| IBIS file stm32f7x2_lqfp176.ibs
[IBIS ver] 4.2
[File name] stm32f7x2_lqfp176.ibs
[File Rev] 1.1
[Date]  21-12-2016
[Source] Data Created at STMicroelectronics
[Notes]  File originated from ELDO simulations.
[Disclaimer]  This information is for modeling purpose only and is
   not guaranted.
   The information is subject to change without notice.
[Copyright] Copyright 2017 STMicroelectronics Inc.
|   Component stm32f7x2_lqfp176
[Component] stm32f7x2_lqfp176
[Manufacturer] STMicroelectronics
[Package]
| variable   typ   min   max
R_pkg   0.0   0.0   0.0
L_pkg   0.0H   0.0H   0.0H
C_pkg   0.0F   0.0F   0.0F
[Pin]  signal_name   model_name   R_pin   L_pin   C_pin
1 PE2 io8p_arsudq_ft 235.000E-3 11.500E-9 327.000E-15
2 PE3 io8p_arsudq_ft 229.900E-3 11.200E-9 303.300E-15
3 PE4 io8p_arsudq_ft 225.000E-3 10.800E-9 280.800E-15
4 PE5 io8p_arsudq_ft 220.400E-3 10.500E-9 259.500E-15
5 PE6 io8p_arsudq_ft 216.000E-3 10.300E-9 239.300E-15
6 VBAT power 211.900E-3 10.000E-9 220.200E-15
7 PI8 io8p_arsudq_ft_v33 208.100E-3 9.700E-9 202.300E-15
8 PC13 io8p_arwsudq_ft_v33 204.400E-3 9.500E-9 185.600E-15
9 PC14-OSC32_IN io8p_arwsudq_ft_v33 201.100E-3 9.300E-9 170.000E-15
10 PC15-OSC32_OUT io8p_arwsudq_ft 198.000E-3 9.100E-9 155.600E-15
11 PI9 io8p_arsudq_ft 195.100E-3 8.900E-9 142.300E-15
12 PI10 io8p_arsudq_ft 192.500E-3 8.700E-9 130.200E-15
13 PI11 io8p_arsudq_ft_v33 190.100E-3 8.600E-9 119.200E-15
14 VSS gnd 188.000E-3 8.400E-9 109.400E-15
15 VDD power 186.100E-3 8.300E-9 100.800E-15
16 PF0 io8p_arsudq_i2c_ft 184.500E-3 8.200E-9 93.300E-15
17 PF1 io8p_arsudq_i2c_ft 183.100E-3 8.100E-9 86.900E-15
18 PF2 io8p_arsudq_ft 182.000E-3 8.000E-9 81.700E-15
19 PF3 io8p_arwsudq_ft 181.100E-3 8.000E-9 77.700E-15
20 PF4 io8p_arwsudq_ft 180.500E-3 7.900E-9 74.800E-15
21 PF5 io8p_arwsudq_ft 180.100E-3 7.900E-9 73.100E-15
22 VSS gnd 180.000E-3 7.900E-9 72.500E-15
23 VDD power 180.000E-3 7.900E-9 72.500E-15
24 PF6 io8p_arwsudq_ft 180.100E-3 7.900E-9 73.100E-15
25 PF7 io8p_arwsudq_ft 180.500E-3 7.900E-9 74.800E-15
26 PF8 io8p_arwsudq_ft 181.100E-3 8.000E-9 77.700E-15
27 PF9 io8p_arwsudq_ft 182.000E-3 8.000E-9 81.700E-15
28 PF10 io8p_arwsudq_ft 183.100E-3 8.100E-9 86.900E-15
29 PH0-OSC_IN io8p_arsudq_ft 184.500E-3 8.200E-9 93.300E-15
30 PH1-OSC_OUT io8p_arsudq_ft 186.100E-3 8.300E-9 100.800E-15
31 NRST ioreset_ft_v33 188.000E-3 8.400E-9 109.400E-15
32 PC0 io8p_ar3wsudq_ft 190.100E-3 8.600E-9 119.200E-15
33 PC1 io8p_ar3wsudq_ft_v33 192.500E-3 8.700E-9 130.200E-15
34 PC2 io8p_ar3wsudq_ft 195.100E-3 8.900E-9 142.300E-15
35 PC3 io8p_ar3wsudq_ft 198.000E-3 9.100E-9 155.600E-15
36 VDD power 201.100E-3 9.300E-9 170.000E-15
37 VSSA gnd 204.400E-3 9.500E-9 185.600E-15
38 VREF+ power 208.100E-3 9.700E-9 202.300E-15
39 VDDA power 211.900E-3 10.000E-9 220.200E-15
40 PA0-WKUP io8p_ar3wsudq_ft_v33 216.000E-3 10.300E-9 239.300E-15
41 PA1 io8p_ar3wsudq_ft 220.400E-3 10.500E-9 259.500E-15
42 PA2 io8p_ar3wsudq_ft_v33 225.000E-3 10.800E-9 280.800E-15
43 PH2 io8p_arsudq_ft 229.900E-3 11.200E-9 303.300E-15
44 PH3 io8p_arsudq_ft 235.000E-3 11.500E-9 327.000E-15
45 PH4 io8p_arsudq_i2c_ft 235.000E-3 11.500E-9 327.000E-15
46 PH5 io8p_arsudq_i2c_ft 229.900E-3 11.200E-9 303.300E-15
47 PA3 io8p_ar3wsudq_ft 225.000E-3 10.800E-9 280.800E-15
48 BYPASS_REG gnd 220.400E-3 10.500E-9 259.500E-15
49 VDD power 216.000E-3 10.300E-9 239.300E-15
50 PA4 io8p_ar3wsudq_ft 211.900E-3 10.000E-9 220.200E-15
51 PA5 io8p_ar3wsudq_ft 208.100E-3 9.700E-9 202.300E-15
52 PA6 io8p_ar3wsudq_ft 204.400E-3 9.500E-9 185.600E-15
53 PA7 io8p_ar3wsudq_ft 201.100E-3 9.300E-9 170.000E-15
54 PC4 io8p_ar3wsudq_ft 198.000E-3 9.100E-9 155.600E-15
55 PC5 io8p_ar3wsudq_ft 195.100E-3 8.900E-9 142.300E-15
56 PB0 io8p_ar3wsudq_ft 192.500E-3 8.700E-9 130.200E-15
57 PB1 io8p_ar3wsudq_ft 190.100E-3 8.600E-9 119.200E-15
58 PB2 io8p_ar3wsudq_ft 188.000E-3 8.400E-9 109.400E-15
59 PF11 io8p_arsudq_ft 186.100E-3 8.300E-9 100.800E-15
60 PF12 io8p_arsudq_ft 184.500E-3 8.200E-9 93.300E-15
61 VSS gnd 183.100E-3 8.100E-9 86.900E-15
62 VDD power 182.000E-3 8.000E-9 81.700E-15
63 PF13 io8p_arsudq_ft 181.100E-3 8.000E-9 77.700E-15
64 PF14 io8p_arsudq_ft 180.500E-3 7.900E-9 74.800E-15
65 PF15 io8p_arsudq_ft 180.100E-3 7.900E-9 73.100E-15
66 PG0 io8p_arsudq_ft 180.000E-3 7.900E-9 72.500E-15
67 PG1 io8p_arsudq_ft 180.000E-3 7.900E-9 72.500E-15
68 PE7 io8p_arsudq_ft 180.100E-3 7.900E-9 73.100E-15
69 PE8 io8p_arsudq_ft 180.500E-3 7.900E-9 74.800E-15
70 PE9 io8p_arsudq_ft 181.100E-3 8.000E-9 77.700E-15
71 VSS gnd 182.000E-3 8.000E-9 81.700E-15
72 VDD power 183.100E-3 8.100E-9 86.900E-15
73 PE10 io8p_arsudq_ft 184.500E-3 8.200E-9 93.300E-15
74 PE11 io8p_arsudq_ft 186.100E-3 8.300E-9 100.800E-15
75 PE12 io8p_arsudq_ft 188.000E-3 8.400E-9 109.400E-15
76 PE13 io8p_arsudq_ft 190.100E-3 8.600E-9 119.200E-15
77 PE14 io8p_arsudq_ft 192.500E-3 8.700E-9 130.200E-15
78 PE15 io8p_ar3wsudq_ft 195.100E-3 8.900E-9 142.300E-15
79 PB10 io8p_arsudq_i2c_ft 198.000E-3 9.100E-9 155.600E-15
80 PB11 io8p_arsudq_i2c_ft 201.100E-3 9.300E-9 170.000E-15
81 VCAP_1 power 204.400E-3 9.500E-9 185.600E-15
82 VDD power 208.100E-3 9.700E-9 202.300E-15
83 PH6 io8p_arsudq_ft 211.900E-3 10.000E-9 220.200E-15
84 PH7 io8p_arsudq_i2c_ft 216.000E-3 10.300E-9 239.300E-15
85 PH8 io8p_arsudq_i2c_ft 220.400E-3 10.500E-9 259.500E-15
86 PH9 io8p_arsudq_ft 225.000E-3 10.800E-9 280.800E-15
87 PH10 io8p_arsudq_ft 229.900E-3 11.200E-9 303.300E-15
88 PH11 io8p_arsudq_ft 235.000E-3 11.500E-9 327.000E-15
89 PH12 io8p_arsudq_ft 235.000E-3 11.500E-9 327.000E-15
90 VSS gnd 229.900E-3 11.200E-9 303.300E-15
91 VDD power 225.000E-3 10.800E-9 280.800E-15
92 PB12 io8usb_id_otg_ft 220.400E-3 10.500E-9 259.500E-15
93 PB13 io8usb_vbus_otg_ft 216.000E-3 10.300E-9 239.300E-15
94 PB14 io8usb_lsfs_otg_ft 211.900E-3 10.000E-9 220.200E-15
95 PB15 io8usb_lsfs_otg_ft 208.100E-3 9.700E-9 202.300E-15
96 PD8 io8p_arsudq_ft 204.400E-3 9.500E-9 185.600E-15
97 PD9 io8p_arsudq_ft 201.100E-3 9.300E-9 170.000E-15
98 PD10 io8p_arsudq_ft 198.000E-3 9.100E-9 155.600E-15
99 PD11 io8p_arsudq_ft 195.100E-3 8.900E-9 142.300E-15
100 PD12 io8p_arsudq_ft 192.500E-3 8.700E-9 130.200E-15
101 PD13 io8p_arsudq_ft 190.100E-3 8.600E-9 119.200E-15
102 VSS gnd 188.000E-3 8.400E-9 109.400E-15
103 VDD power 186.100E-3 8.300E-9 100.800E-15
104 PD14 io8p_arsudq_ft 184.500E-3 8.200E-9 93.300E-15
105 PD15 io8p_arsudq_ft 183.100E-3 8.100E-9 86.900E-15
106 PG2 io8p_arsudq_ft 182.000E-3 8.000E-9 81.700E-15
107 PG3 io8p_arsudq_ft 181.100E-3 8.000E-9 77.700E-15
108 PG4 io8p_arsudq_ft 180.500E-3 7.900E-9 74.800E-15
109 PG5 io8p_arsudq_ft 180.100E-3 7.900E-9 73.100E-15
110 PG6 io8p_arsudq_ft 180.000E-3 7.900E-9 72.500E-15
111 PG7 io8p_arsudq_ft 180.000E-3 7.900E-9 72.500E-15
112 PG8 io8p_arsudq_ft 180.100E-3 7.900E-9 73.100E-15
113 VSS gnd 180.500E-3 7.900E-9 74.800E-15
114 VDDUSB power 181.100E-3 8.000E-9 77.700E-15
115 PC6 io8p_arsudq_ft 182.000E-3 8.000E-9 81.700E-15
116 PC7 io8p_arsudq_ft 183.100E-3 8.100E-9 86.900E-15
117 PC8 io8p_arsudq_ft 184.500E-3 8.200E-9 93.300E-15
118 PC9 io8p_arsudq_i2c_ft 186.100E-3 8.300E-9 100.800E-15
119 PA8 io8p_arsudq_i2c_ft 188.000E-3 8.400E-9 109.400E-15
120 PA9 io8usb_vbus_otg_ft 190.100E-3 8.600E-9 119.200E-15
121 PA10 io8usb_id_otg_ft 192.500E-3 8.700E-9 130.200E-15
122 PA11 io8usb_lsfs_otg_ft 195.100E-3 8.900E-9 142.300E-15
123 PA12 io8usb_lsfs_otg_ft 198.000E-3 9.100E-9 155.600E-15
124 PA13 io8p_arsudq_ft 201.100E-3 9.300E-9 170.000E-15
125 VCAP_2 power 204.400E-3 9.500E-9 185.600E-15
126 VSS gnd 208.100E-3 9.700E-9 202.300E-15
127 VDD power 211.900E-3 10.000E-9 220.200E-15
128 PH13 io8p_arsudq_ft 216.000E-3 10.300E-9 239.300E-15
129 PH14 io8p_arsudq_ft 220.400E-3 10.500E-9 259.500E-15
130 PH15 io8p_arsudq_ft 225.000E-3 10.800E-9 280.800E-15
131 PI0 io8p_arsudq_ft 229.900E-3 11.200E-9 303.300E-15
132 PI1 io8p_arsudq_ft 235.000E-3 11.500E-9 327.000E-15
133 PI2 io8p_arsudq_ft 235.000E-3 11.500E-9 327.000E-15
134 PI3 io8p_arsudq_ft 229.900E-3 11.200E-9 303.300E-15
135 VSS gnd 225.000E-3 10.800E-9 280.800E-15
136 VDD power 220.400E-3 10.500E-9 259.500E-15
137 PA14 io8p_arsudq_ft 216.000E-3 10.300E-9 239.300E-15
138 PA15 io8p_arsudq_ft 211.900E-3 10.000E-9 220.200E-15
139 PC10 io8p_arsudq_ft 208.100E-3 9.700E-9 202.300E-15
140 PC11 io8p_arsudq_ft 204.400E-3 9.500E-9 185.600E-15
141 PC12 io8p_arsudq_ft 201.100E-3 9.300E-9 170.000E-15
142 PD0 io8p_arsudq_ft 198.000E-3 9.100E-9 155.600E-15
143 PD1 io8p_arsudq_ft 195.100E-3 8.900E-9 142.300E-15
144 PD2 io8p_arsudq_ft 192.500E-3 8.700E-9 130.200E-15
145 PD3 io8p_arsudq_ft 190.100E-3 8.600E-9 119.200E-15
146 PD4 io8p_arsudq_ft 188.000E-3 8.400E-9 109.400E-15
147 PD5 io8p_arsudq_ft 186.100E-3 8.300E-9 100.800E-15
148 VSS gnd 184.500E-3 8.200E-9 93.300E-15
149 VDDSDMMC power 183.100E-3 8.100E-9 86.900E-15
150 PD6 io8p_arsudq_ft 182.000E-3 8.000E-9 81.700E-15
151 PD7 io8p_arsudq_ft 181.100E-3 8.000E-9 77.700E-15
152 PG9 io8p_arsudq_ft 180.500E-3 7.900E-9 74.800E-15
153 PG10 io8p_arsudq_ft 180.100E-3 7.900E-9 73.100E-15
154 PG11 io8p_arsudq_ft 180.000E-3 7.900E-9 72.500E-15
155 PG12 io8p_arsudq_ft 180.000E-3 7.900E-9 72.500E-15
156 PG13 io8p_arsudq_ft 180.100E-3 7.900E-9 73.100E-15
157 PG14 io8p_arsudq_ft 180.500E-3 7.900E-9 74.800E-15
158 VSS gnd 181.100E-3 8.000E-9 77.700E-15
159 VDD power 182.000E-3 8.000E-9 81.700E-15
160 PG15 io8p_arsudq_ft 183.100E-3 8.100E-9 86.900E-15
161 PB3 io8p_arsudq_ft 184.500E-3 8.200E-9 93.300E-15
162 PB4 io8p_arsudq_ft 186.100E-3 8.300E-9 100.800E-15
163 PB5 io8p_ar3wsudq_ft 188.000E-3 8.400E-9 109.400E-15
164 PB6 io8p_arsudq_i2c_ft 190.100E-3 8.600E-9 119.200E-15
165 PB7 io8p_arsudq_i2c_ft 192.500E-3 8.700E-9 130.200E-15
166 BOOT0 vpp_test_hv 195.100E-3 8.900E-9 142.300E-15
167 PB8 io8p_arsudq_i2c_ft 198.000E-3 9.100E-9 155.600E-15
168 PB9 io8p_arsudq_i2c_ft 201.100E-3 9.300E-9 170.000E-15
169 PE0 io8p_arsudq_ft 204.400E-3 9.500E-9 185.600E-15
170 PE1 io8p_arsudq_ft 208.100E-3 9.700E-9 202.300E-15
171 PDR_ON gnd 211.900E-3 10.000E-9 220.200E-15
172 VDD power 216.000E-3 10.300E-9 239.300E-15
173 PI4 io8p_arsudq_ft 220.400E-3 10.500E-9 259.500E-15
174 PI5 io8p_arsudq_ft 225.000E-3 10.800E-9 280.800E-15
175 PI6 io8p_arsudq_ft 229.900E-3 11.200E-9 303.300E-15
176 PI7 io8p_arsudq_ft 235.000E-3 11.500E-9 327.000E-15
[Diff Pin]   inv_pin   vdiff   tdelay_typ  tdelay_min  tdelay_max
94   95   NA   NA   NA   NA
122   123   NA   NA   NA   NA
[Model Selector] io8p_arsudq_ft_v33
io8p00_arsudq_ft_v33_pd_lv  "SPEED00 1P8V, PD=40kOhm"
io8p00_arsudq_ft_v33_pu_lv  "SPEED00 1P8V, PU=40kOhm"
io8p00_arsudq_ft_v33_lv  "SPEED00 1P8V"
io8p01_arsudq_ft_v33_pd_lv  "SPEED01 1P8V, PD=40kOhm"
io8p01_arsudq_ft_v33_pu_lv  "SPEED01 1P8V, PU=40kOhm"
io8p01_arsudq_ft_v33_lv  "SPEED01 1P8V"
io8p10_arsudq_ft_v33_pd_lv  "SPEED10 1P8V, PD=40kOhm"
io8p10_arsudq_ft_v33_pu_lv  "SPEED10 1P8V, PU=40kOhm"
io8p10_arsudq_ft_v33_lv  "SPEED10 1P8V"
io8p11_arsudq_ft_v33_pd_lv  "SPEED11 1P8V, PD=40kOhm"
io8p11_arsudq_ft_v33_pu_lv  "SPEED11 1P8V, PU=40kOhm"
io8p11_arsudq_ft_v33_lv  "SPEED11 1P8V"
io8p00_arsudq_ft_v33_pd  "SPEED00, PD=40kOhm"
io8p00_arsudq_ft_v33_pu  "SPEED00, PU=40kOhm"
io8p00_arsudq_ft_v33  "SPEED00"
io8p01_arsudq_ft_v33_pd  "SPEED01, PD=40kOhm"
io8p01_arsudq_ft_v33_pu  "SPEED01, PU=40kOhm"
io8p01_arsudq_ft_v33  "SPEED01"
io8p10_arsudq_ft_v33_pd  "SPEED10, PD=40kOhm"
io8p10_arsudq_ft_v33_pu  "SPEED10, PU=40kOhm"
io8p10_arsudq_ft_v33  "SPEED10"
io8p11_arsudq_ft_v33_pd  "SPEED11, PD=40kOhm"
io8p11_arsudq_ft_v33_pu  "SPEED11, PU=40kOhm"
io8p11_arsudq_ft_v33  "SPEED11"
[Model Selector] io8p_ar3wsudq_ft
io8p00_ar3wsudq_ft_pd_lv  "SPEED00 1P8V, PD=40kOhm"
io8p00_ar3wsudq_ft_pu_lv  "SPEED00 1P8V, PU=40kOhm"
io8p00_ar3wsudq_ft_lv  "SPEED00 1P8V"
io8p01_ar3wsudq_ft_pd_lv  "SPEED01 1P8V, PD=40kOhm"
io8p01_ar3wsudq_ft_pu_lv  "SPEED01 1P8V, PU=40kOhm"
io8p01_ar3wsudq_ft_lv  "SPEED01 1P8V"
io8p10_ar3wsudq_ft_pd_lv  "SPEED10 1P8V, PD=40kOhm"
io8p10_ar3wsudq_ft_pu_lv  "SPEED10 1P8V, PU=40kOhm"
io8p10_ar3wsudq_ft_lv  "SPEED10 1P8V"
io8p11_ar3wsudq_ft_pd_lv  "SPEED11 1P8V, PD=40kOhm"
io8p11_ar3wsudq_ft_pu_lv  "SPEED11 1P8V, PU=40kOhm"
io8p11_ar3wsudq_ft_lv  "SPEED11 1P8V"
io8p00_ar3wsudq_ft_pd  "SPEED00, PD=40kOhm"
io8p00_ar3wsudq_ft_pu  "SPEED00, PU=40kOhm"
io8p00_ar3wsudq_ft  "SPEED00"
io8p01_ar3wsudq_ft_pd  "SPEED01, PD=40kOhm"
io8p01_ar3wsudq_ft_pu  "SPEED01, PU=40kOhm"
io8p01_ar3wsudq_ft  "SPEED01"
io8p10_ar3wsudq_ft_pd  "SPEED10, PD=40kOhm"
io8p10_ar3wsudq_ft_pu  "SPEED10, PU=40kOhm"
io8p10_ar3wsudq_ft  "SPEED10"
io8p11_ar3wsudq_ft_pd  "SPEED11, PD=40kOhm"
io8p11_ar3wsudq_ft_pu  "SPEED11, PU=40kOhm"
io8p11_ar3wsudq_ft  "SPEED11"
[Model Selector] io8p_ar3wsudq_ft_v33
io8p00_ar3wsudq_ft_v33_pd_lv  "SPEED00 1P8V, PD=40kOhm"
io8p00_ar3wsudq_ft_v33_pu_lv  "SPEED00 1P8V, PU=40kOhm"
io8p00_ar3wsudq_ft_v33_lv  "SPEED00 1P8V"
io8p01_ar3wsudq_ft_v33_pd_lv  "SPEED01 1P8V, PD=40kOhm"
io8p01_ar3wsudq_ft_v33_pu_lv  "SPEED01 1P8V, PU=40kOhm"
io8p01_ar3wsudq_ft_v33_lv  "SPEED01 1P8V"
io8p10_ar3wsudq_ft_v33_pd_lv  "SPEED10 1P8V, PD=40kOhm"
io8p10_ar3wsudq_ft_v33_pu_lv  "SPEED10 1P8V, PU=40kOhm"
io8p10_ar3wsudq_ft_v33_lv  "SPEED10 1P8V"
io8p11_ar3wsudq_ft_v33_pd_lv  "SPEED11 1P8V, PD=40kOhm"
io8p11_ar3wsudq_ft_v33_pu_lv  "SPEED11 1P8V, PU=40kOhm"
io8p11_ar3wsudq_ft_v33_lv  "SPEED11 1P8V"
io8p00_ar3wsudq_ft_v33_pd  "SPEED00, PD=40kOhm"
io8p00_ar3wsudq_ft_v33_pu  "SPEED00, PU=40kOhm"
io8p00_ar3wsudq_ft_v33  "SPEED00"
io8p01_ar3wsudq_ft_v33_pd  "SPEED01, PD=40kOhm"
io8p01_ar3wsudq_ft_v33_pu  "SPEED01, PU=40kOhm"
io8p01_ar3wsudq_ft_v33  "SPEED01"
io8p10_ar3wsudq_ft_v33_pd  "SPEED10, PD=40kOhm"
io8p10_ar3wsudq_ft_v33_pu  "SPEED10, PU=40kOhm"
io8p10_ar3wsudq_ft_v33  "SPEED10"
io8p11_ar3wsudq_ft_v33_pd  "SPEED11, PD=40kOhm"
io8p11_ar3wsudq_ft_v33_pu  "SPEED11, PU=40kOhm"
io8p11_ar3wsudq_ft_v33  "SPEED11"
[Model Selector] io8p_arsudq_ft
io8p00_arsudq_ft_pd_lv  "SPEED00 1P8V, PD=40kOhm"
io8p00_arsudq_ft_pu_lv  "SPEED00 1P8V, PU=40kOhm"
io8p00_arsudq_ft_lv  "SPEED00 1P8V"
io8p01_arsudq_ft_pd_lv  "SPEED01 1P8V, PD=40kOhm"
io8p01_arsudq_ft_pu_lv  "SPEED01 1P8V, PU=40kOhm"
io8p01_arsudq_ft_lv  "SPEED01 1P8V"
io8p10_arsudq_ft_pd_lv  "SPEED10 1P8V, PD=40kOhm"
io8p10_arsudq_ft_pu_lv  "SPEED10 1P8V, PU=40kOhm"
io8p10_arsudq_ft_lv  "SPEED10 1P8V"
io8p11_arsudq_ft_pd_lv  "SPEED11 1P8V, PD=40kOhm"
io8p11_arsudq_ft_pu_lv  "SPEED11 1P8V, PU=40kOhm"
io8p11_arsudq_ft_lv  "SPEED11 1P8V"
io8p00_arsudq_ft_pd  "SPEED00, PD=40kOhm"
io8p00_arsudq_ft_pu  "SPEED00, PU=40kOhm"
io8p00_arsudq_ft  "SPEED00"
io8p01_arsudq_ft_pd  "SPEED01, PD=40kOhm"
io8p01_arsudq_ft_pu  "SPEED01, PU=40kOhm"
io8p01_arsudq_ft  "SPEED01"
io8p10_arsudq_ft_pd  "SPEED10, PD=40kOhm"
io8p10_arsudq_ft_pu  "SPEED10, PU=40kOhm"
io8p10_arsudq_ft  "SPEED10"
io8p11_arsudq_ft_pd  "SPEED11, PD=40kOhm"
io8p11_arsudq_ft_pu  "SPEED11, PU=40kOhm"
io8p11_arsudq_ft  "SPEED11"
[Model Selector] io8p_arsudq_i2c_ft
io8prog_1v8_i2c_pd  "5V Tol GPIO 1.8V range i2c functionality with pull down"
io8prog_1v8_i2c_pu  "5V Tol GPIO 1.8V range i2c functionality with pull up"
io8prog_1v8_i2c  "5V Tol GPIO 1.8V range i2c functionality"
io8prog_3v3_i2c_pd  "5V Tol GPIO 3.3V range i2c functionality with pull down"
io8prog_3v3_i2c_pu  "5V Tol GPIO 3.3V range i2c functionality with pull up"
io8prog_3v3_i2c  "5V Tol GPIO 3.3V range i2c functionality"
io8prog_1v8_pd_00  "5V Tol GPIO 1.8V range with pd speed 00"
io8prog_1v8_pu_00  "5V Tol GPIO 1.8V range with pu speed 00"
io8prog_1v8_00  "5V Tol GPIO 1.8V range speed 00"
io8prog_3v3_pd_00  "5V Tol GPIO 3.3V range with pd speed 00"
io8prog_3v3_pu_00  "5V Tol GPIO 3.3V range with pu speed 00"
io8prog_3v3_00  "5V Tol GPIO 3.3V range speed 00"
io8prog_1v8_pd_01  "5V Tol GPIO 1.8V range with pd speed 01"
io8prog_1v8_pu_01  "5V Tol GPIO 1.8V range with pu speed 01"
io8prog_1v8_01  "5V Tol GPIO 1.8V range speed 01"
io8prog_3v3_pd_01  "5V Tol GPIO 3.3V range with pd speed 01"
io8prog_3v3_pu_01  "5V Tol GPIO 3.3V range with pu speed 01"
io8prog_3v3_01  "5V Tol GPIO 3.3V range speed 01"
io8prog_1v8_pd_10  "5V Tol GPIO 1.8V range with pd speed 10"
io8prog_1v8_pu_10  "5V Tol GPIO 1.8V range with pu speed 10"
io8prog_1v8_10  "5V Tol GPIO 1.8V range speed 10"
io8prog_3v3_pd_10  "5V Tol GPIO 3.3V range with pd speed 10"
io8prog_3v3_pu_10  "5V Tol GPIO 3.3V range with pu speed 10"
io8prog_3v3_10  "5V Tol GPIO 3.3V range speed 10"
io8prog_1v8_pd_11  "5V Tol GPIO 1.8V range with pd speed 11"
io8prog_1v8_pu_11  "5V Tol GPIO 1.8V range with pu speed 11"
io8prog_1v8_11  "5V Tol GPIO 1.8V range speed 11"
io8prog_3v3_pd_11  "5V Tol GPIO 3.3V range with pd speed 11"
io8prog_3v3_pu_11  "5V Tol GPIO 3.3V range with pu speed 11"
io8prog_3v3_11  "5V Tol GPIO 3.3V range speed 11"
[Model Selector] io8p_arwsudq_ft
io8p00_arwsudq_ft_pd_lv  "SPEED00 1P8V, PD=40kOhm"
io8p00_arwsudq_ft_pu_lv  "SPEED00 1P8V, PU=40kOhm"
io8p00_arwsudq_ft_lv  "SPEED00 1P8V"
io8p01_arwsudq_ft_pd_lv  "SPEED01 1P8V, PD=40kOhm"
io8p01_arwsudq_ft_pu_lv  "SPEED01 1P8V, PU=40kOhm"
io8p01_arwsudq_ft_lv  "SPEED01 1P8V"
io8p10_arwsudq_ft_pd_lv  "SPEED10 1P8V, PD=40kOhm"
io8p10_arwsudq_ft_pu_lv  "SPEED10 1P8V, PU=40kOhm"
io8p10_arwsudq_ft_lv  "SPEED10 1P8V"
io8p11_arwsudq_ft_pd_lv  "SPEED11 1P8V, PD=40kOhm"
io8p11_arwsudq_ft_pu_lv  "SPEED11 1P8V, PU=40kOhm"
io8p11_arwsudq_ft_lv  "SPEED11 1P8V"
io8p00_arwsudq_ft_pd  "SPEED00, PD=40kOhm"
io8p00_arwsudq_ft_pu  "SPEED00, PU=40kOhm"
io8p00_arwsudq_ft  "SPEED00"
io8p01_arwsudq_ft_pd  "SPEED01, PD=40kOhm"
io8p01_arwsudq_ft_pu  "SPEED01, PU=40kOhm"
io8p01_arwsudq_ft  "SPEED01"
io8p10_arwsudq_ft_pd  "SPEED10, PD=40kOhm"
io8p10_arwsudq_ft_pu  "SPEED10, PU=40kOhm"
io8p10_arwsudq_ft  "SPEED10"
io8p11_arwsudq_ft_pd  "SPEED11, PD=40kOhm"
io8p11_arwsudq_ft_pu  "SPEED11, PU=40kOhm"
io8p11_arwsudq_ft  "SPEED11"
[Model Selector] io8p_arwsudq_ft_v33
io8p00_arwsudq_ft_v33_pd_lv  "SPEED00 1P8V, PD=40kOhm"
io8p00_arwsudq_ft_v33_pu_lv  "SPEED00 1P8V, PU=40kOhm"
io8p00_arwsudq_ft_v33_lv  "SPEED00 1P8V"
io8p01_arwsudq_ft_v33_pd_lv  "SPEED01 1P8V, PD=40kOhm"
io8p01_arwsudq_ft_v33_pu_lv  "SPEED01 1P8V, PU=40kOhm"
io8p01_arwsudq_ft_v33_lv  "SPEED01 1P8V"
io8p10_arwsudq_ft_v33_pd_lv  "SPEED10 1P8V, PD=40kOhm"
io8p10_arwsudq_ft_v33_pu_lv  "SPEED10 1P8V, PU=40kOhm"
io8p10_arwsudq_ft_v33_lv  "SPEED10 1P8V"
io8p11_arwsudq_ft_v33_pd_lv  "SPEED11 1P8V, PD=40kOhm"
io8p11_arwsudq_ft_v33_pu_lv  "SPEED11 1P8V, PU=40kOhm"
io8p11_arwsudq_ft_v33_lv  "SPEED11 1P8V"
io8p00_arwsudq_ft_v33_pd  "SPEED00, PD=40kOhm"
io8p00_arwsudq_ft_v33_pu  "SPEED00, PU=40kOhm"
io8p00_arwsudq_ft_v33  "SPEED00"
io8p01_arwsudq_ft_v33_pd  "SPEED01, PD=40kOhm"
io8p01_arwsudq_ft_v33_pu  "SPEED01, PU=40kOhm"
io8p01_arwsudq_ft_v33  "SPEED01"
io8p10_arwsudq_ft_v33_pd  "SPEED10, PD=40kOhm"
io8p10_arwsudq_ft_v33_pu  "SPEED10, PU=40kOhm"
io8p10_arwsudq_ft_v33  "SPEED10"
io8p11_arwsudq_ft_v33_pd  "SPEED11, PD=40kOhm"
io8p11_arwsudq_ft_v33_pu  "SPEED11, PU=40kOhm"
io8p11_arwsudq_ft_v33  "SPEED11"
[Model Selector] io8usb_id_otg_ft
io8p00_id_otg_ft_pd_lv  "SPEED00 1P8V, PD=14kOhm"
io8p00_id_otg_ft_pu_lv  "SPEED00 1P8V, PU=14kOhm"
io8p00_id_otg_ft_lv  "SPEED00 1P8V"
io8p01_id_otg_ft_pd_lv  "SPEED01 1P8V, PD=14kOhm"
io8p01_id_otg_ft_pu_lv  "SPEED01 1P8V, PU=14kOhm"
io8p01_id_otg_ft_lv  "SPEED01 1P8V"
io8p10_id_otg_ft_pd_lv  "SPEED10 1P8V, PD=14kOhm"
io8p10_id_otg_ft_pu_lv  "SPEED10 1P8V, PU=14kOhm"
io8p10_id_otg_ft_lv  "SPEED10 1P8V"
io8p11_id_otg_ft_pd_lv  "SPEED11 1P8V, PD=14kOhm"
io8p11_id_otg_ft_pu_lv  "SPEED11 1P8V, PU=14kOhm"
io8p11_id_otg_ft_lv  "SPEED11 1P8V"
io8p00_id_otg_ft_pd  "SPEED00, PD=14kOhm"
io8p00_id_otg_ft_pu  "SPEED00, PU=14kOhm"
io8p00_id_otg_ft  "SPEED00"
io8p01_id_otg_ft_pd  "SPEED01, PD=14kOhm"
io8p01_id_otg_ft_pu  "SPEED01, PU=14kOhm"
io8p01_id_otg_ft  "SPEED01"
io8p10_id_otg_ft_pd  "SPEED10, PD=14kOhm"
io8p10_id_otg_ft_pu  "SPEED10, PU=14kOhm"
io8p10_id_otg_ft  "SPEED10"
io8p11_id_otg_ft_pd  "SPEED11, PD=14kOhm"
io8p11_id_otg_ft_pu  "SPEED11, PU=14kOhm"
io8p11_id_otg_ft  "SPEED11"
[Model Selector] io8usb_lsfs_otg_ft
io8usb_ls_otg_ft_dpdn_pd  "LS USB DP/DN IO + PD=20kOhm"
io8usb_ls_otg_ft_dpdn_pupu2  "LS USB DP/DN IO + PU/PU2=2.2kOhm"
io8usb_ls_otg_ft_dpdn_pu2  "LS USB DP/DN IO + PU2=1.2kOhm"
io8usb_ls_otg_ft_dpdn_pu  "LS USB DP/DN IO + PU=1.2kOhm"
io8usb_ls_otg_ft_dpdn  "LS USB DP/DN IO"
io8usb_fs_otg_ft_dpdn_pd  "HS USB DP/DN IO + PD=20kOhm"
io8usb_fs_otg_ft_dpdn_pupu2  "HS USB DP/DN IO + PU/PU2=2.2kOhm"
io8usb_fs_otg_ft_dpdn_pu2  "HS USB DP/DN IO + PU2=1.2kOhm"
io8usb_fs_otg_ft_dpdn_pu  "HS USB DP/DN IO + PU=1.2kOhm"
io8usb_fs_otg_ft_dpdn  "HS USB DP/DN IO"
io8p00_lsfs_otg_ft_pd_lv  "SPEED00 1P8V, PD=40kOhm"
io8p00_lsfs_otg_ft_pu_lv  "SPEED00 1P8V, PU=40kOhm"
io8p00_lsfs_otg_ft_lv  "SPEED00 1P8V"
io8p01_lsfs_otg_ft_pd_lv  "SPEED01 1P8V, PD=40kOhm"
io8p01_lsfs_otg_ft_pu_lv  "SPEED01 1P8V, PU=40kOhm"
io8p01_lsfs_otg_ft_lv  "SPEED01 1P8V"
io8p10_lsfs_otg_ft_pd_lv  "SPEED10 1P8V, PD=40kOhm"
io8p10_lsfs_otg_ft_pu_lv  "SPEED10 1P8V, PU=40kOhm"
io8p10_lsfs_otg_ft_lv  "SPEED10 1P8V"
io8p11_lsfs_otg_ft_pd_lv  "SPEED11 1P8V, PD=40kOhm"
io8p11_lsfs_otg_ft_pu_lv  "SPEED11 1P8V, PU=40kOhm"
io8p11_lsfs_otg_ft_lv  "SPEED11 1P8V"
io8p00_lsfs_otg_ft_pd  "SPEED00, PD=40kOhm"
io8p00_lsfs_otg_ft_pu  "SPEED00, PU=40kOhm"
io8p00_lsfs_otg_ft  "SPEED00"
io8p01_lsfs_otg_ft_pd  "SPEED01, PD=40kOhm"
io8p01_lsfs_otg_ft_pu  "SPEED01, PU=40kOhm"
io8p01_lsfs_otg_ft  "SPEED01"
io8p10_lsfs_otg_ft_pd  "SPEED10, PD=40kOhm"
io8p10_lsfs_otg_ft_pu  "SPEED10, PU=40kOhm"
io8p10_lsfs_otg_ft  "SPEED10"
io8p11_lsfs_otg_ft_pd  "SPEED11, PD=40kOhm"
io8p11_lsfs_otg_ft_pu  "SPEED11, PU=40kOhm"
io8p11_lsfs_otg_ft  "SPEED11"
[Model Selector] io8usb_vbus_otg_ft
io8psenb_vbus_otg_ft  "VBUS PULSE, SENSE VB"
io8psenab_vbus_otg_ft  "VBUS PULSE, SENSE VA and VB"
io8psena_vbus_otg_ft  "VBUS PULSE, SENSE VA"
io8psen_vbus_otg_ft  "VBUS PULSE"
io8p00_vbus_otg_ft_pd_lv  "SPEED00 1P8V, PD=40kOhm"
io8p00_vbus_otg_ft_pu_lv  "SPEED00 1P8V, PU=40kOhm"
io8p00_vbus_otg_ft_lv  "SPEED00 1P8V"
io8p01_vbus_otg_ft_pd_lv  "SPEED01 1P8V, PD=40kOhm"
io8p01_vbus_otg_ft_pu_lv  "SPEED01 1P8V, PU=40kOhm"
io8p01_vbus_otg_ft_lv  "SPEED01 1P8V"
io8p10_vbus_otg_ft_pd_lv  "SPEED10 1P8V, PD=40kOhm"
io8p10_vbus_otg_ft_pu_lv  "SPEED10 1P8V, PU=40kOhm"
io8p10_vbus_otg_ft_lv  "SPEED10 1P8V"
io8p11_vbus_otg_ft_pd_lv  "SPEED11 1P8V, PD=40kOhm"
io8p11_vbus_otg_ft_pu_lv  "SPEED11 1P8V, PU=40kOhm"
io8p11_vbus_otg_ft_lv  "SPEED11 1P8V"
io8p00_vbus_otg_ft_pd  "SPEED00, PD=40kOhm"
io8p00_vbus_otg_ft_pu  "SPEED00, PU=40kOhm"
io8p00_vbus_otg_ft  "SPEED00"
io8p01_vbus_otg_ft_pd  "SPEED01, PD=40kOhm"
io8p01_vbus_otg_ft_pu  "SPEED01, PU=40kOhm"
io8p01_vbus_otg_ft  "SPEED01"
io8p10_vbus_otg_ft_pd  "SPEED10, PD=40kOhm"
io8p10_vbus_otg_ft_pu  "SPEED10, PU=40kOhm"
io8p10_vbus_otg_ft  "SPEED10"
io8p11_vbus_otg_ft_pd  "SPEED11, PD=40kOhm"
io8p11_vbus_otg_ft_pu  "SPEED11, PU=40kOhm"
io8p11_vbus_otg_ft  "SPEED11"
[Model Selector] ioreset_ft_v33
ioreset_ft_v33_pu_lv  "IORESET 1P8V + PU=40kOhm"
ioreset_ft_v33_nopu_lv  "IORESET 1P8V"
ioreset_ft_v33_pu  "IORESET + PU=40kOhm"
ioreset_ft_v33_nopu  "IORESET"
[Model Selector] vpp_test_hv
vpp_test_hv_2p4  "Input Buffer 1P8V"
vpp_test_hv_3p3  "Input Buffer"
| Models and submodels in the file (266): io8p00_arsudq_ft_v33_pd_lv (I/O), io8p00_arsudq_ft_v33_pu_lv (I/O), io8p00_arsudq_ft_v33_lv (I/O), io8p01_arsudq_ft_v33_pd_lv (I/O), io8p01_arsudq_ft_v33_pu_lv (I/O), io8p01_arsudq_ft_v33_lv (I/O), io8p10_arsudq_ft_v33_pd_lv (I/O), io8p10_arsudq_ft_v33_pu_lv (I/O), io8p10_arsudq_ft_v33_lv (I/O), io8p11_arsudq_ft_v33_pd_lv (I/O), io8p11_arsudq_ft_v33_pu_lv (I/O), io8p11_arsudq_ft_v33_lv (I/O), io8p00_arsudq_ft_v33_pd (I/O), io8p00_arsudq_ft_v33_pu (I/O), io8p00_arsudq_ft_v33 (I/O), io8p01_arsudq_ft_v33_pd (I/O), io8p01_arsudq_ft_v33_pu (I/O), io8p01_arsudq_ft_v33 (I/O), io8p10_arsudq_ft_v33_pd (I/O), io8p10_arsudq_ft_v33_pu (I/O), io8p10_arsudq_ft_v33 (I/O), io8p11_arsudq_ft_v33_pd (I/O), io8p11_arsudq_ft_v33_pu (I/O), io8p11_arsudq_ft_v33 (I/O), io8p00_ar3wsudq_ft_pd_lv (I/O), io8p00_ar3wsudq_ft_pu_lv (I/O), io8p00_ar3wsudq_ft_lv (I/O), io8p01_ar3wsudq_ft_pd_lv (I/O), io8p01_ar3wsudq_ft_pu_lv (I/O), io8p01_ar3wsudq_ft_lv (I/O), io8p10_ar3wsudq_ft_pd_lv (I/O), io8p10_ar3wsudq_ft_pu_lv (I/O), io8p10_ar3wsudq_ft_lv (I/O), io8p11_ar3wsudq_ft_pd_lv (I/O), io8p11_ar3wsudq_ft_pu_lv (I/O), io8p11_ar3wsudq_ft_lv (I/O), io8p00_ar3wsudq_ft_pd (I/O), io8p00_ar3wsudq_ft_pu (I/O), io8p00_ar3wsudq_ft (I/O), io8p01_ar3wsudq_ft_pd (I/O), io8p01_ar3wsudq_ft_pu (I/O), io8p01_ar3wsudq_ft (I/O), io8p10_ar3wsudq_ft_pd (I/O), io8p10_ar3wsudq_ft_pu (I/O), io8p10_ar3wsudq_ft (I/O), io8p11_ar3wsudq_ft_pd (I/O), io8p11_ar3wsudq_ft_pu (I/O), io8p11_ar3wsudq_ft (I/O), io8p00_ar3wsudq_ft_v33_pd_lv (I/O), io8p00_ar3wsudq_ft_v33_pu_lv (I/O), io8p00_ar3wsudq_ft_v33_lv (I/O), io8p01_ar3wsudq_ft_v33_pd_lv (I/O), io8p01_ar3wsudq_ft_v33_pu_lv (I/O), io8p01_ar3wsudq_ft_v33_lv (I/O), io8p10_ar3wsudq_ft_v33_pd_lv (I/O), io8p10_ar3wsudq_ft_v33_pu_lv (I/O), io8p10_ar3wsudq_ft_v33_lv (I/O), io8p11_ar3wsudq_ft_v33_pd_lv (I/O), io8p11_ar3wsudq_ft_v33_pu_lv (I/O), io8p11_ar3wsudq_ft_v33_lv (I/O), io8p00_ar3wsudq_ft_v33_pd (I/O), io8p00_ar3wsudq_ft_v33_pu (I/O), io8p00_ar3wsudq_ft_v33 (I/O), io8p01_ar3wsudq_ft_v33_pd (I/O), io8p01_ar3wsudq_ft_v33_pu (I/O), io8p01_ar3wsudq_ft_v33 (I/O), io8p10_ar3wsudq_ft_v33_pd (I/O), io8p10_ar3wsudq_ft_v33_pu (I/O), io8p10_ar3wsudq_ft_v33 (I/O), io8p11_ar3wsudq_ft_v33_pd (I/O), io8p11_ar3wsudq_ft_v33_pu (I/O), io8p11_ar3wsudq_ft_v33 (I/O), io8p00_arsudq_ft_pd_lv (I/O), io8p00_arsudq_ft_pu_lv (I/O), io8p00_arsudq_ft_lv (I/O), io8p01_arsudq_ft_pd_lv (I/O), io8p01_arsudq_ft_pu_lv (I/O), io8p01_arsudq_ft_lv (I/O), io8p10_arsudq_ft_pd_lv (I/O), io8p10_arsudq_ft_pu_lv (I/O)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
